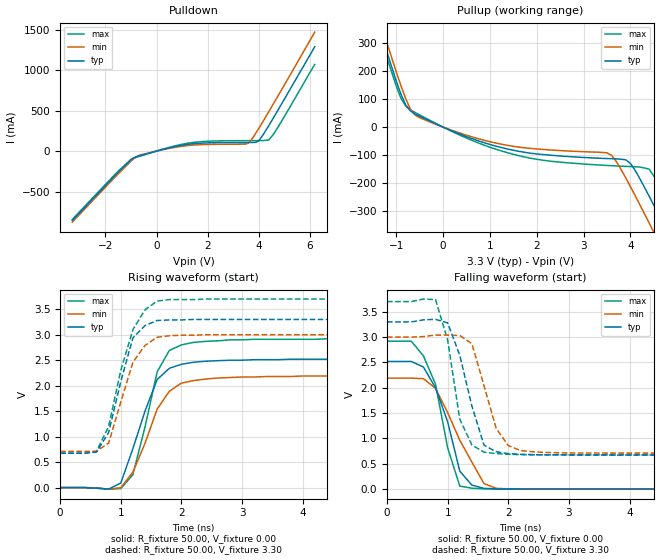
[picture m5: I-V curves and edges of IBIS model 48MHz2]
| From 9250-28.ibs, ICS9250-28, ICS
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|   Model 48MHz2
[Model]   48MHz2
Model_type   Output
Polarity   Non-Inverting
Vmeas = 1.5V
Cref = 20pF
Rref = 0
Vref = 1.5V
C_comp   5.50pF   5.00pF   6.00pF
[Temperature Range]   27.00   70.00   0.00
[Voltage Range]   3.30V   3.00V   3.70V
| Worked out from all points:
|   slope of the pulldown table from 0 to 0.495 V, typ, clamps not added: 12.4 ohm
|   slope of the pullup table from 0 to 0.495 V, typ, clamps not added: 14.7 ohm
|   rising waveform, R_fixture 50.00, V_fixture 0.00: 20-80 % time 444ps typ, 474ps min, 361ps max; typ from 0 V to 2.52 V
|   rising waveform, R_fixture 50.00, V_fixture 3.30: 20-80 % time 338ps typ, 377ps min, 384ps max; typ from 0.674 V to 3.3 V
|   falling waveform, R_fixture 50.00, V_fixture 0.00: 20-80 % time 377ps typ, 546ps min, 357ps max; typ from 2.52 V to 0 V
|   falling waveform, R_fixture 50.00, V_fixture 3.30: 20-80 % time 356ps typ, 339ps min, 278ps max; typ from 3.3 V to 0.674 V
[Pulldown]
| voltage   I(typ)   I(min)   I(max)
-3.3V     -857.9mA   -878.4mA   -845.3mA
-1.5V     -261.3mA   -282.1mA   -248.7mA
-1V       -107.9mA   -125mA     -102.2mA
-700mV    -61.18mA   -54.61mA   -68.48mA
400mV     32.81mA    27.49mA    37.39mA
1.3V      86.08mA    70.47mA    101mA
3.6V      106.5mA    98.57mA    128.8mA
3.9V      108.8mA    225.9mA    129.5mA
4V        126.6mA    276.5mA    129.7mA
4.4V      314.9mA    487.2mA    137.4mA
4.8V      527.7mA    703mA      316.3mA
6.2V      1.29A      1.47A      1.07A
[Pullup]
| voltage   I(typ)   I(min)   I(max)
-3.3V     1.4A       1.43A      1.38A
-1.5V     421.2mA    455.2mA    400.3mA
-900mV    116.5mA    146.2mA    102mA
-700mV    57.52mA    63.85mA    61.81mA
-500mV    38.48mA    33.44mA    43.28mA
1.4V      -78.79mA   -65.56mA   -92.19mA
3.5V      -111.7mA   -91.56mA   -136.3mA
4V        -128.7mA   -211.2mA   -140.2mA
4.4V      -245.1mA   -340.5mA   -149.2mA
4.8V      -375.8mA   -472.8mA   -260.1mA
5.2V      -509mA     -606.4mA   -391.1mA
6.2V      -845.7mA   -943.1mA   -726.8mA
[Ramp]
| variable   typ   min   max
dV/dt_r   1.51/354.04p   1.31/416.22p   1.75/312.34p
dV/dt_f   1.58/300.00p   1.37/300.00p   1.81/300.00p
[Rising Waveform]
R_fixture = 50.00
V_fixture = 0.00
V_fixture_min = 0.00
V_fixture_max = 0.00
| time   V(typ)   V(min)   V(max)
0s        0V         0V         0V
800ps     -31.01mV   -29.88mV   -31.17mV
1ns       89.14mV    -3.03mV    -19.9mV
1.2ns     765.6mV    303mV      254mV
1.4ns     1.5V       870.1mV    1.19V
1.6ns     2.12V      1.54V      2.27V
1.8ns     2.34V      1.89V      2.69V
2ns       2.42V      2.05V      2.8V
3.4ns     2.51V      2.18V      2.91V
10ns      2.52V      2.19V      2.92V
[Rising Waveform]
R_fixture = 50.00
V_fixture = 3.30
V_fixture_min = 3.00
V_fixture_max = 3.70
| time   V(typ)   V(min)   V(max)
0s        673.6mV    711.3mV    675.9mV
400ps     673.6mV    711.3mV    675.9mV
600ps     696.8mV    712.9mV    712.6mV
800ps     1.08V      874mV      1.2V
1ns       2.08V      1.68V      2.3V
1.2ns     2.94V      2.46V      3.1V
1.4ns     3.18V      2.79V      3.49V
1.6ns     3.28V      2.95V      3.66V
2.4ns     3.3V       3V         3.7V
10ns      3.3V       3V         3.7V
[Falling Waveform]
R_fixture = 50.00
V_fixture = 0.00
V_fixture_min = 0.00
V_fixture_max = 0.00
| time   V(typ)   V(min)   V(max)
0s        2.52V      2.19V      2.92V
400ps     2.52V      2.19V      2.92V
600ps     2.41V      2.18V      2.63V
800ps     2V         1.99V      2.07V
1ns       1.33V      1.51V      817.2mV
1.2ns     355.4mV    965.6mV    60.84mV
1.4ns     79.4mV     534.8mV    19.11mV
1.6ns     15.91mV    109mV      7.22mV
1.8ns     6.17mV     16.27mV    3.69mV
10ns      0V         1.56uV     652.7nV
[Falling Waveform]
R_fixture = 50.00
V_fixture = 3.30
V_fixture_min = 3.00
V_fixture_max = 3.70
| time   V(typ)   V(min)   V(max)
0s        3.3V       3V         3.7V
800ps     3.35V      3.04V      3.74V
1ns       3.28V      3.04V      2.94V
1.2ns     2.64V      3.03V      1.38V
1.4ns     1.64V      2.87V      871.5mV
1.6ns     866.9mV    2.04V      731.3mV
1.8ns     737.7mV    1.2V       700.7mV
2ns       701.1mV    861.1mV    687.7mV
2.2ns     687.2mV    761.6mV    681.9mV
10ns      673.6mV    711.3mV    675.9mV
